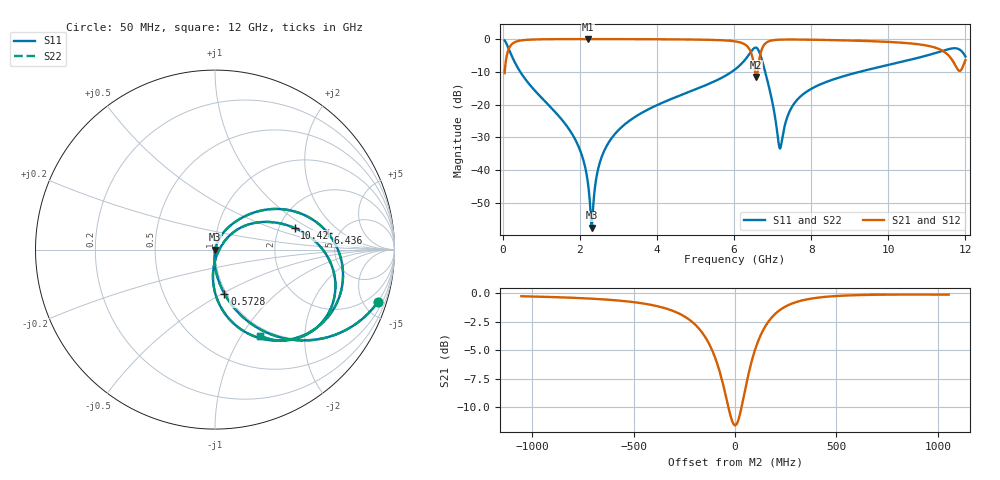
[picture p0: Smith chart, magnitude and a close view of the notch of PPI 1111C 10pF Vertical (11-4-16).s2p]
# GHz S MA R 50
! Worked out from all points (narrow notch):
!   1601 points, 50 MHz to 12 GHz, reference 50 ohm
!   highest |S21| = -0.01 dB at 2.216 GHz (marker M1); lowest = -11.6 dB at 6.578 GHz (marker M2)
!   notch at M2: 11.3 dB deep, 176 MHz wide at half that depth
!   lowest |S11| = -57.5 dB at 2.306 GHz (marker M3), VSWR 1.00, Z = 50.1 - j0.0404 ohm
!   |S11| at or under -10 dB: 456.2 MHz to 5.94 GHz (5.483 GHz wide, 171 % of centre); 6.807 GHz to 9.254 GHz (2.446 GHz wide, 30.5 % of centre)
!   |S22| runs from -57.5 to -0.4 dB; largest |S21 - S12| = 0
!   S11 on the Smith chart (normalised r, x): 50 MHz: 0.98, -6.23; 572.8 MHz: 0.98, -0.51; 6.436 GHz: 4.06, +1.27; 10.42 GHz: 2.43, +0.74; 12 GHz: 0.89, -1.21
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0.05  0.9533 -17.8  0.3019 72.2  0.3019 72.2  0.9533 -17.8
0.2665938  0.5047 -60.9  0.8628 29.1  0.8628 29.1  0.5047 -60.9
0.5728125  0.2513 -78.0  0.9672 11.9  0.9672 11.9  0.2513 -78.0
2.044156  0.01758 -94.5  0.9985 -8.5  0.9985 -8.5  0.01758 -94.5
2.215937  0.006067 -87.7  0.9986 -10.0  0.9986 -10.0  0.006067 -87.7
2.305563  0.001333 -17.6  0.9985 -10.7  0.9985 -10.7  0.001333 -17.6
2.492281  0.01145 70.8  0.9984 -12.3  0.9984 -12.3  0.01145 70.8
2.753687  0.02677 72.5  0.998 -14.3  0.998 -14.3  0.02677 72.5
4.038312  0.1005 64.4  0.9926 -24.4  0.9926 -24.4  0.1005 64.4
6.025  0.3438 39.6  0.922 -47.6  0.922 -47.6  0.3438 39.6
6.435781  0.635 8.4  0.631 -67.3  0.631 -67.3  0.635 8.4
6.577687  0.7375 -28.1  0.2635 -35.1  0.2635 -35.1  0.7375 -28.1
6.674781  0.5896 -58.9  0.558 0.0  0.558 0.0  0.5896 -58.9
6.80175  0.3256 -84.0  0.8452 -12.9  0.8452 -12.9  0.3256 -84.0
7.190125  0.02143 -26.1  0.9783 -32.7  0.9783 -32.7  0.02143 -26.1
7.496344  0.09122 43.4  0.9834 -39.0  0.9834 -39.0  0.09122 43.4
8.019156  0.1764 41.3  0.9762 -46.2  0.9762 -46.2  0.1764 41.3
10.01331  0.4048 20.6  0.9041 -68.0  0.9041 -68.0  0.4048 20.6
10.41662  0.4598 15.2  0.8737 -73.1  0.8737 -73.1  0.4598 15.2
11.59669  0.7095 -19.3  0.5349 -93.3  0.5349 -93.3  0.7095 -19.3
11.83569  0.6987 -42.2  0.328 -70.6  0.328 -70.6  0.6987 -42.2
12  0.5406 -62.4  0.4785 -39.8  0.4785 -39.8  0.5406 -62.4
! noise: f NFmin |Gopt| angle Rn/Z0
0.05  0.0003708  0.8718  2.028  0.0006232
1.372  0.003676  0.6682  6.774  0.002121
2.701  0.00618  0.6244  12.42  0.003043
4.031  0.008967  0.6196  17.96  0.004294
5.36  0.01532  0.6953  23.76  0.009412
6.682  0.1684  0.9607  30.39  0.9024
8.012  0.02359  0.7132  35.39  0.01477
9.341  0.02478  0.6942  40.09  0.01401
10.67  0.04425  0.7982  45.84  0.0386
12  0.314  0.9659  51.79  1.69
